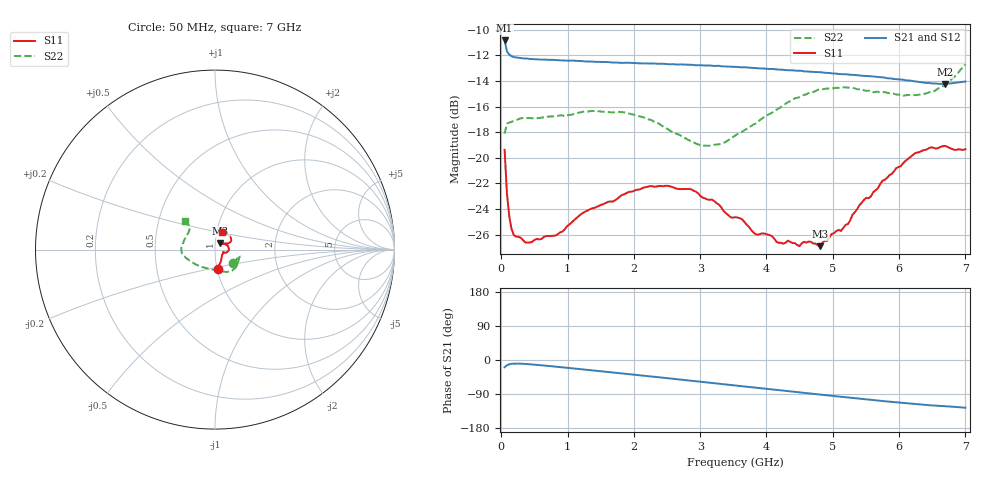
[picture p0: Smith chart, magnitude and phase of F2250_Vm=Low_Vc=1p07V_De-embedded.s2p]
! Integrated Device Technology
! Corporate Headquarters
! 6024 Silver Creek Valley Road
! San Jose, CA 95138  USA
! Phone:  1-408-284-8200
! Toll Free:  1-800-223-1366
! Webpage:  http://www.idt.com/
! Timing and RF Division
! 515 Groton Road, Suite 102
! Westford, MA 01886-6024
! Device:  F2250
! Description: Voltage Variable RF Attenuator
! Frequency:  50.0 -  6000.00 MHz
! Package:  3x3 mm Thin QFN Plastic Package: 16 pin
! Ports:  2 RF, 3 DC
!  Pin  1  = GND
!  Pin  2  = NC
!  Pin  3  = RF1  = Port 1
!  Pin  4  = NC
!  Pin  5  = GND
!  Pin  6  = GND
!  Pin  7  = GND
!  Pin  8  = GND
!  Pin  9  = NC
!  Pin 10  = RF2  = Port 2
!  Pin 11  = NC
!  Pin 12  = GND
!  Pin 13  = GND
!  Pin 14  = VCNTRL
!  Pin 15  = VDD
!  Pin 16  = VMODE
! Vcntrl:  1.070 Volts
! Vmode:  +0.000 Volts
! Vdd:  +3.30  Volts
! Current:  1.188 mA
! Data:  The device was measured on a the F2250 evaluation board which has
!  individual transmission lines to the RF pins.  Data was collected
!  using a calibrated network analyzer.  The evaluation board was
!  de-embedded using a TRL calibration technique.
!  The reference plane is the edge of the package pin.
! Misc:  SN 10
!  Action Tracker AT0258
! Date Measured:  2014-11-26
! Date:  2015-10-15  MJV
! Note:
!  Integrated Device Technology supplies this data as a sample of measured
!  data at the package pin for this product.  Your particular data for this
!  product may vary.
!  Data was taken at 25 degrees C.
!  Integrated Device Technology reserves the right to change this data at anytime.
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# GHz S dB R 50
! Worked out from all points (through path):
!   201 points, 50 MHz to 7 GHz, reference 50 ohm
!   highest |S21| = -10.85 dB at 50 MHz (marker M1); lowest = -14.3 dB at 6.687 GHz (marker M2)
!   group delay of S21, straight-line fit = 49.8 ps
!   lowest |S11| = -26.9 dB at 4.811 GHz (marker M3), VSWR 1.09, Z = 52.8 + j3.68 ohm
!   |S11| at or under -10 dB: start of sweep to end of sweep
!   |S22| runs from -19.1 to -12.7 dB; largest |S21 - S12| = 0.00075
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0.05  -19.38 -82.5  -10.85 -19.1  -10.85 -19.1  -18.12 -35.8
0.08475  -22.75 -63.0  -11.69 -13.8  -11.69 -13.8  -17.34 -19.9
0.1195  -24.53 -52.2  -11.95 -11.4  -11.96 -11.4  -17.26 -15.2
0.189  -26.03 -37.5  -12.15 -9.7  -12.14 -9.7  -17.12 -13.4
0.3975  -26.62 -21.5  -12.26 -10.8  -12.27 -10.8  -16.90 -15.8
0.8145  -26.07 -17.0  -12.37 -17.4  -12.38 -17.4  -16.75 -28.5
1.2315  -24.30 -16.9  -12.47 -24.8  -12.47 -24.8  -16.41 -39.8
1.857  -22.83 -8.6  -12.59 -36.0  -12.57 -36.1  -16.45 -53.1
2.37825  -22.20 1.4  -12.67 -45.6  -12.65 -45.6  -17.33 -65.7
2.86475  -22.46 14.3  -12.74 -54.7  -12.75 -54.7  -18.71 -86.5
3.0385  -23.11 19.6  -12.79 -58.0  -12.78 -58.0  -19.05 -96.7
3.525  -24.64 35.3  -12.90 -67.2  -12.90 -67.2  -18.27 -127.6
3.83775  -25.97 47.6  -13.00 -73.0  -13.00 -73.0  -17.32 -143.5
4.18525  -26.63 56.5  -13.12 -79.5  -13.12 -79.5  -16.15 -157.8
4.7065  -26.69 55.2  -13.30 -89.3  -13.30 -89.3  -14.86 -171.5
4.81075  -26.89 50.3  -13.32 -91.2  -13.33 -91.2  -14.65 -173.4
5.22775  -25.17 36.1  -13.50 -98.9  -13.49 -98.9  -14.52 177.4
5.471  -23.27 29.9  -13.61 -103.2  -13.60 -103.2  -14.74 171.9
5.85325  -21.36 25.1  -13.81 -109.9  -13.78 -110.0  -14.96 161.8
6.2355  -19.66 29.1  -14.04 -116.2  -14.05 -116.3  -15.11 149.3
6.68725  -19.07 45.4  -14.25 -121.8  -14.23 -121.9  -14.27 137.0
7  -19.33 68.1  -14.05 -126.0  -14.03 -126.1  -12.71 136.9
